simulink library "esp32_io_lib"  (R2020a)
settings: Solver=VariableStepAuto  StartTime=0.0  StopTime=10.0  RelTol=1e-3
undefined symbols (not defined in the file): Advanced, DigitalInput, DigitalOutput, Disable, empty, ESP_INTR_FLAG_LEVEL2, GPIO_DRIVE_CAP_2, GPIO_FLOATING, GPIO_INTR_ANYEDGE, GPIO_MODE_INPUT_OUTPUT, GPIOInterrupt, Level, NULL

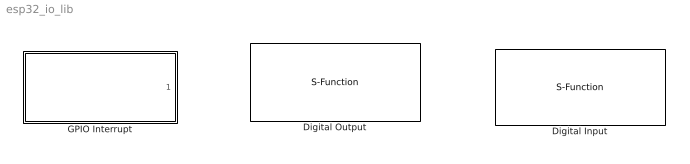
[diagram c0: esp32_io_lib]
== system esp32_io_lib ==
  Digital Input : S-Function  FunctionName=esp32_digital_input  Parameters=blockid,sampletime,pull_mode_define,pin0,pin1,pin2,pin3,pin4,pin5,pin6,pin7,pin8,pin9,pin10,pin11,pin12,pin13,pin14,pin15,pin16,pin17,pin18,pin19,pin20,pin21,pin22,pin23,pin24,pin25,pin26,pin27,pin28,pin29,pin30,pin31,pin32,pin33,pin34,pin35,pin36,pin37,pin38,pin39,pin40,pin41,pin42,pin43,pin44,pin45,pin46,pin47,pin48,pin_hold_define,deep_sleep_pin_hold_define,pin_string,pin_array,numpins  SFunctionDeploymentMode=off  EnableBusSupport=off  mask(esp32_digital_input){blockid=DigitalInput, settings=Advanced, overridepin=off, pin0=off, pin1=off, pin2=off, pin3=off, pin4=off, pin5=off, pin6=off, pin7=off, pin8=off, pin9=off, pin10=off, pin11=off, pin12=off, pin13=off, pin14=off, pin15=off, pin16=on, pin17=off, pin18=off, pin19=off, pin20=off, pin21=off, pin22=off, pin23=off, pin24=off, pin25=off, pin26=off, pin27=off, pin28=off, pin29=off, pin30=off, pin31=off, pin32=off, pin33=off, pin34=off, pin35=off, pin36=off, pin37=off, pin38=off, pin39=off, pin40=off, pin41=off, pin42=off, pin43=off, pin44=off, pin45=off, pin46=off, pin47=off, pin48=off, pull_mode=None (floating), pin_hold=Disable, deep_sleep_pin_hold=Disable, pin_array=[0  0  0  0  0  0  0  0  0  0  0  0  0  0  0  0  1  0  0  0  0  0  0  0  0  0  0  0  0  0  0  0  0  0  0  0  0  0  0  0  0  0  0  0  0  0  0  0  0], inport_num=1, pin_hold_define=off, pull_mode_define=GPIO_FLOATING, deep_sleep_pin_hold_define=off, pin_string=((1ULL<<16)), numpins=49, sampletime=-1}
      mask prompts: settings "Settings interface:"; overridepin "Override pin selection constraints"; pin0 "Pin 0"; pin1 "Pin 1"; pin2 "Pin 2"; pin3 "Pin 3"; pin4 "Pin 4"; pin5 "Pin 5"; pin6 "Pin 6"; pin7 "Pin 7"; pin8 "Pin 8"; pin9 "Pin 9"; pin10 "Pin 10"; pin11 "Pin 11"; pin12 "Pin 12"; pin13 "Pin 13"; pin14 "Pin 14"; pin15 "Pin 15"; pin16 "Pin 16"; pin17 "Pin 17"; pin18 "Pin 18"; pin19 "Pin 19"; pin20 "Pin 20"; pin21 "Pin 21"; pin22 "Pin 22"; pin23 "Pin 23"; pin24 "Pin 24"; pin25 "Pin 25"; pin26 "Pin 26"; pin27 "Pin 27"; pin28 "Pin 28"; pin29 "Pin 29"; pin30 "Pin 30"; pin31 "Pin 31"; pin32 "Pin 32"; pin33 "Pin 33"; pin34 "Pin 34"; pin35 "Pin 35"; pin36 "Pin 36"; pin37 "Pin 37"; pin38 "Pin 38"; pin39 "Pin 39"; pin40 "Pin 40"; pin41 "Pin 41"; pin42 "Pin 42"; pin43 "Pin 43"; pin44 "Pin 44"; pin45 "Pin 45"; pin46 "Pin 46"; pin47 "Pin 47"; pin48 "Pin 48"; pull_mode "pull mode:"; pin_hold "Pin hold:"; deep_sleep_pin_hold "Deep sleep pin hold (affects all GPIO):"; pin_array "Pin array"; inport_num "Input_ports"; pin_hold_define "Def pin hold"; pull_mode_define "Def pull mode"; deep_sleep_pin_hold_define "Def pin hold sleep"; pin_string "Pin String"; sampletime "Sample time (sec)"
      mask help: Digital Input pin block for ESP32. The pins can be configured with 'Basic' and 'Advanced' settings. In 'Basic' settings, the pin is configured with no pull-up/pull-down resistors and no 'pin hold' functionality In 'Advanced' settings, the user has the full control over the configured GPIO out pins.
      mask init:
      | esp32_digital_input_callback('init');
  Digital Output : S-Function  FunctionName=esp32_digital_output  Parameters=blockid,sampletime,pin_mode_define,pin0,pin1,pin2,pin3,pin4,pin5,pin6,pin7,pin8,pin9,pin10,pin11,pin12,pin13,pin14,pin15,pin16,pin17,pin18,pin19,pin20,pin21,pin22,pin23,pin24,pin25,pin26,pin27,pin28,pin29,pin30,pin31,pin32,pin33,pin34,pin35,pin36,pin37,pin38,pin39,pin40,pin41,pin42,pin43,pin44,pin45,pin46,pin47,pin48,drive_capability_define,pin_hold_define,deep_sleep_pin_hold_define,pin_string,pin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  SFunctionDeploymentMode=off  EnableBusSupport=off  mask(esp32_digital_output){blockid=DigitalOutput, settings=Advanced, overridepin=off, pin0=off, pin1=off, pin2=on, pin3=off, pin4=off, pin5=off, pin6=off, pin7=off, pin8=off, pin9=off, pin10=off, pin11=off, pin12=off, pin13=off, pin14=off, pin15=off, pin16=off, pin17=off, pin18=off, pin19=off, pin20=off, pin21=off, pin22=off, pin23=off, pin24=off, pin25=off, pin26=off, pin27=off, pin28=off, pin29=off, pin30=off, pin31=off, pin32=off, pin33=off, pin34=off, pin35=off, pin36=off, pin37=off, pin38=off, pin39=off, pin40=off, pin41=off, pin42=off, pin43=off, pin44=off, pin45=off, pin46=off, pin47=off, pin48=off, pin_initialize=on, pin_mode=Push-pull, sampletime=-1, drive_capability=Normal (default), pin_hold=Disable, deep_sleep_pin_hold=Disable, pin_array=[0  0  1  0  0  0  0  0  0  0  0  0  0  0  0  0  0  0  0  0  0  0  0  0  0  0  0  0  0  0  0  0  0  0  0  0  0  0  0  0  0  0  0  0  0  0  0  0  0], inport_num=1, drive_capability_define=GPIO_DRIVE_CAP_2, pin_hold_define=off, pin_mode_define=GPIO_MODE_INPUT_OUTPUT, deep_sleep_pin_hold_define=off, pin_string=((1ULL<<2)), numpins=49}
      mask prompts: settings "Settings interface:"; overridepin "Override pin selection constraints"; pin0 "Pin 0"; pin1 "Pin 1"; pin2 "Pin 2"; pin3 "Pin 3"; pin4 "Pin 4"; pin5 "Pin 5"; pin6 "Pin 6"; pin7 "Pin 7"; pin8 "Pin 8"; pin9 "Pin 9"; pin10 "Pin 10"; pin11 "Pin 11"; pin12 "Pin 12"; pin13 "Pin 13"; pin14 "Pin 14"; pin15 "Pin 15"; pin16 "Pin 16"; pin17 "Pin 17"; pin18 "Pin 18"; pin19 "Pin 19"; pin20 "Pin 20"; pin21 "Pin 21"; pin22 "Pin 22"; pin23 "Pin 23"; pin24 "Pin 24"; pin25 "Pin 25"; pin26 "Pin 26"; pin27 "Pin 27"; pin28 "Pin 28"; pin29 "Pin 29"; pin30 "Pin 30"; pin31 "Pin 31"; pin32 "Pin 32"; pin33 "Pin 33"; pin34 "Pin 34"; pin35 "Pin 35"; pin36 "Pin 36"; pin37 "Pin 37"; pin38 "Pin 38"; pin39 "Pin 39"; pin40 "Pin 40"; pin41 "Pin 41"; pin42 "Pin 42"; pin43 "Pin 43"; pin44 "Pin 44"; pin45 "Pin 45"; pin46 "Pin 46"; pin47 "Pin 47"; pin48 "Pin 48"; pin_initialize "Initialize the above pins"; pin_mode "Pin mode:"; sampletime "Sample time (sec)"; drive_capability "Drive capability:"; pin_hold "Pin hold:"; deep_sleep_pin_hold "Deep sleep pin hold (affects all GPIO):"; pin_array "Pin array"; inport_num "Input_ports"; drive_capability_define "Def drive capability"; pin_hold_define "Def pin hold"; pin_mode_define "Def pin mode"; deep_sleep_pin_hold_define "Def pin hold sleep"; pin_string "Pin String"
      mask help: Digital output pin block for ESP32. The pins can be configured with 'Basic' and 'Advanced' settings. In 'Basic' settings, the pin mode is push-pull with no 'pin hold' and the pin drive strength is at default. In 'Advanced' settings, the user has the full control over the configured GPIO out pins.
      mask init:
      | esp32_digital_output_callback('init');
  GPIO Interrupt : Subsystem  mask(esp32_gpio_interrupt){pin=0, trigger_type=Both edges, trigger_type_define=GPIO_INTR_ANYEDGE, interrupt_priority=Level 2, interrupt_priority_define=ESP_INTR_FLAG_LEVEL2, blockid=GPIOInterrupt, sampletime=-1, check_destination_block=NULL, destination_is_xTask=empty}
      mask prompts: pin "GPIO pin:"; trigger_type "Trigger type:"; trigger_type_define "Trigger type define"; interrupt_priority "Interrupt priority level:"; interrupt_priority_define "Interrupt priority define"; blockid "Block ID"; sampletime "Sample time (sec)"; check_destination_block "Check destination block"; destination_is_xTask "Destination block type"
      mask help: This block can be used to set up an Interrupt Service Routine (ISR) that could be triggered by an input signal to one of the digital pins.
      mask init:
      | esp32_gpio_interrupt_callback('init');

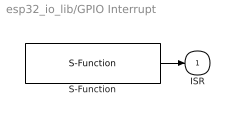
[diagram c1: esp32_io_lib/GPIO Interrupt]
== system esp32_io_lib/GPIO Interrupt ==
  S-Function : S-Function  FunctionName=esp32_gpio_interrupt  Parameters=blockid, sampletime, pin, trigger_type_define, interrupt_priority_define, destination_is_xTask  SFunctionDeploymentMode=off  EnableBusSupport=off
  ISR : Outport  VectorParamsAs1DForOutWhenUnconnected=off
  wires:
  S-Function/1 -> ISR/1
